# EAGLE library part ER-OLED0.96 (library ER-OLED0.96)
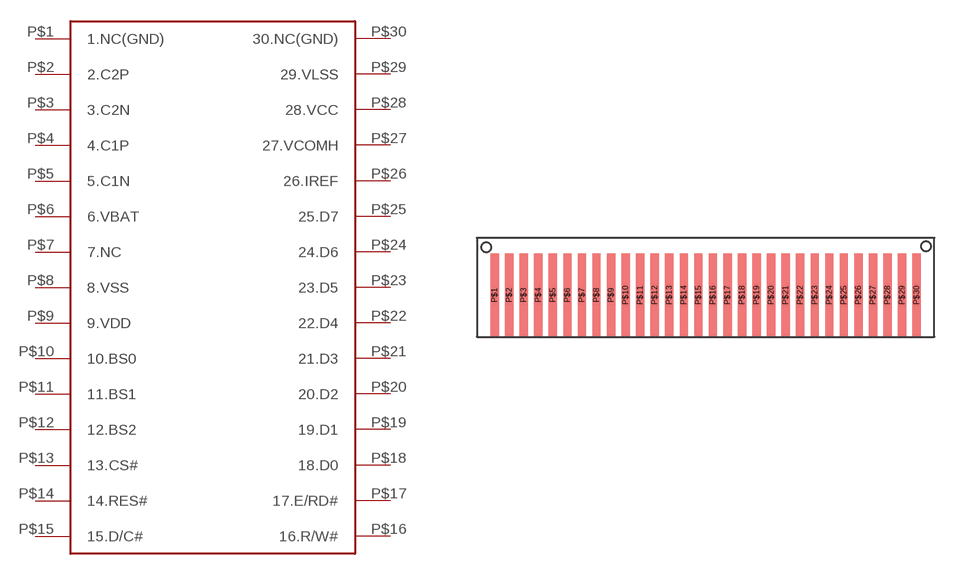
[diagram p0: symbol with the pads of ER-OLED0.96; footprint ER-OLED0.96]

Designator prefix -

## ER-OLED0.96  [ER-OLED0.96]
P$1  1.NC(GND)
P$2  2.C2P
P$3  3.C2N
P$4  4.C1P
P$5  5.C1N
P$6  6.VBAT
P$7  7.NC
P$8  8.VSS
P$9  9.VDD
P$10  10.BS0
P$11  11.BS1
P$12  12.BS2
P$13  13.CS#
P$14  14.RES#
P$15  15.D/C#
P$16  16.R/W#
P$17  17.E/RD#
P$18  18.D0
P$19  19.D1
P$20  20.D2
P$21  21.D3
P$22  22.D4
P$23  23.D5
P$24  24.D6
P$25  25.D7
P$26  26.IREF
P$27  27.VCOMH
P$28  28.VCC
P$29  29.VLSS
P$30  30.NC(GND)

## Footprint ER-OLED0.96 (pad centres in mm)
smd 0.4 x 4: P$1 0.85,2; P$2 1.55,2; P$3 2.25,2; P$4 2.95,2; P$5 3.65,2; P$6 4.35,2; P$7 5.05,2; P$8 5.75,2; P$9 6.45,2; P$10 7.15,2; P$11 7.85,2; P$12 8.55,2; P$13 9.25,2; P$14 9.95,2; P$15 10.65,2; P$16 11.35,2; P$17 12.05,2; P$18 12.75,2; P$19 13.45,2; P$20 14.15,2; P$21 14.85,2; P$22 15.55,2; P$23 16.25,2; P$24 16.95,2; P$25 17.65,2; P$26 18.35,2; P$27 19.05,2; P$28 19.75,2; P$29 20.45,2; P$30 21.15,2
